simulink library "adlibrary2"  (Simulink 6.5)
undefined symbols (not defined in the file or in its folder): adlibrary2, ADM, DDRII, II, no_bitstream, SRAM, SX, XP, XRC
libraries: xbsIndex_r4 x360, adlibrary2 x9, adlibrary2_d2sram_0 x5, adlibrary2_ddr2dram_1 x4, adlibrary2_ddr_xpi0 x4, adlibrary2_ddr_xpl x3, adlibrary2_xpl32 x1, adlibrary2_xpl64 x1, adlibrary2_zbt64 x1, adlibrary2_zbt4_0 x1, adlibrary2_zbt4_1 x1, adlibrary2_zbt4_2 x1
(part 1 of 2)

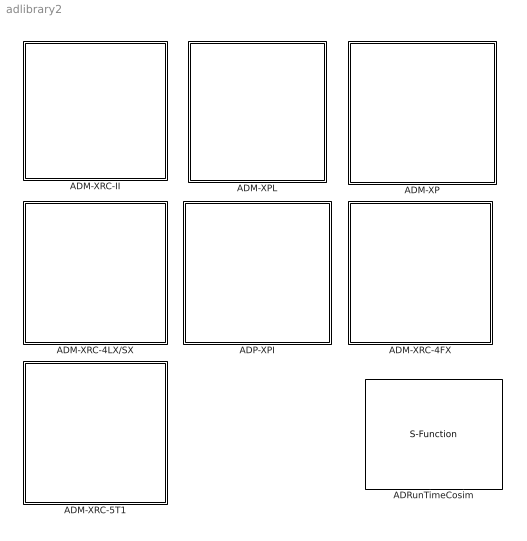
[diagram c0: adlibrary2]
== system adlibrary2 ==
  ADM-XP : Subsystem
  ADM-XPL : Subsystem
  ADM-XRC-4FX : Subsystem  AncestorBlock=adlibrary2/ADM-XRC-4LX//SX
  ADM-XRC-4LX/SX : Subsystem  AncestorBlock=adlibrary2/ADM-XRC-II
  ADM-XRC-5T1 : Subsystem  AncestorBlock=adlibrary2/ADM-XRC-4FX
  ADM-XRC-II : Subsystem
  ADP-XPI : Subsystem
  ADRunTimeCosim : S-Function  FunctionName=adcosim  Parameters='',index,bitstream,freq,single_step,shared  mask{index=0, bitstream=no_bitstream, freq=50, single_step=off, shared=None}
      mask prompts: index "Card Index"; freq "Clock Frequency"; single_step "Single Step"; shared "Share Access"

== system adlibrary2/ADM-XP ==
  DDR SDRAM 0 : Subsystem  mask{memsize=1}
      mask prompts: memsize "Simulation RAM Size (Mb)"
  DDR SDRAM 1 : Subsystem  mask{memsize=1}
      mask prompts: memsize "Simulation RAM Size (Mb)"
  DDRII SRAM 0 : Subsystem  mask{rate=1}
      mask prompts: rate "Simulink Clock Period"
  DDRII SRAM 1 : Subsystem  AncestorBlock=adlibrary2/ADM-XP/DDRII SRAM 0  mask{rate=1}
      mask prompts: rate "Simulink Clock Period"
  DDRII SRAM 2 : Subsystem  mask{rate=1}
      mask prompts: rate "Simulink Clock Period"
  DDRII SRAM 3 : Subsystem  mask{rate=1}
      mask prompts: rate "Simulink Clock Period"
  XPL 32 Bit Interface : adlibrary2/ADM-XPL/XPL 32 Bit Interface  SystemSampleTime=-1  program='load myprogram.txt'  clock_ratio=1.5  sstep_clk_sel_default=0
  XPL 64 Bit Interface : adlibrary2/ADM-XPL/XPL 64 Bit Interface  SystemSampleTime=-1  program='load myprogram.txt'  clock_ratio=1.5  sstep_clk_sel_default=0

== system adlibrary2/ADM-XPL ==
  DDR SDRAM : Subsystem  mask{memsize=1}
      mask prompts: memsize "Simulation RAM Size (Mb)"
  XPL 32 Bit Interface : Subsystem  mask{program='load myprogram.txt', clock_ratio=1.5, sstep_clk_sel_default=0}
      mask prompts: program "Local Bus Script Program"; clock_ratio "Clock Ratio"
  XPL 64 Bit Interface : Subsystem  mask{program='load myprogram.txt', clock_ratio=1.5, sstep_clk_sel_default=0}
      mask prompts: program "Local Bus Script Program"; clock_ratio "Clock Ratio"
  ZBT SRAM 64 : Subsystem  mask{rate=1}
      mask prompts: rate "Simulink Clock Period"

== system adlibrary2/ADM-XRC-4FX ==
  DDRII DRAM 0 : Subsystem  mask{rate=1}
      mask prompts: rate "Simulink Clock Period"
  DDRII DRAM 1 : Subsystem  mask{rate=1}
      mask prompts: rate "Simulink Clock Period"
  DDRII DRAM 2 : Subsystem  mask{rate=1}
      mask prompts: rate "Simulink Clock Period"
  DDRII DRAM 3 : Subsystem  mask{rate=1}
      mask prompts: rate "Simulink Clock Period"
  XPL 32 Bit Interface : adlibrary2/ADM-XPL/XPL 32 Bit Interface  SystemSampleTime=-1  program='load myprogram.txt'  clock_ratio=1.5  sstep_clk_sel_default=0
  XPL 64 Bit Interface : adlibrary2/ADM-XPL/XPL 64 Bit Interface  SystemSampleTime=-1  program='load myprogram.txt'  clock_ratio=1.5  sstep_clk_sel_default=0

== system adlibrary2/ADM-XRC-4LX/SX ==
  PLX 32 Bit Interface : adlibrary2/ADM-XRC-II/PLX 32 Bit Interface  SystemSampleTime=-1  program='load myprogram.txt'  clock_ratio=1.5  sstep_clk_sel_default=0
  ZBT SRAM 0 : Subsystem
  ZBT SRAM 1 : Subsystem
  ZBT SRAM 2 : Subsystem
  ZBT SRAM 3 : Subsystem
  ZBT SRAM 4 : Subsystem
  ZBT SRAM 5 : Subsystem

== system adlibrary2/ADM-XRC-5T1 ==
  DDRII DRAM 0 : Subsystem  mask{rate=1}
      mask prompts: rate "Simulink Clock Period"
  DDRII DRAM 1 : Subsystem  mask{rate=1}
      mask prompts: rate "Simulink Clock Period"
  XPL 32 Bit Interface : adlibrary2/ADM-XPL/XPL 32 Bit Interface  SystemSampleTime=-1  program='load myprogram.txt'  clock_ratio=1.5  sstep_clk_sel_default=0
  XPL 64 Bit Interface : adlibrary2/ADM-XPL/XPL 64 Bit Interface  SystemSampleTime=-1  program='load myprogram.txt'  clock_ratio=1.5  sstep_clk_sel_default=0

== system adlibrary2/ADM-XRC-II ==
  PLX 32 Bit Interface : Subsystem  mask{program='load myprogram.txt', clock_ratio=1.5, sstep_clk_sel_default=0}
      mask prompts: program "Local Bus Script Program"; clock_ratio "Clock Ratio"
  "XRM DDR SDRAM " : Subsystem  mask{memsize=1}
      mask prompts: memsize "Simulation RAM Size (Mb)"
  ZBT SRAM 0 : Subsystem  mask{rate=1}
      mask prompts: rate "Simulink Clock Period"
  ZBT SRAM 1 : Subsystem  mask{rate=1}
      mask prompts: rate "Simulink Clock Period"
  ZBT SRAM 2 : Subsystem  mask{rate=1}
      mask prompts: rate "Simulink Clock Period"
  ZBT SRAM 3 : Subsystem  mask{rate=1}
      mask prompts: rate "Simulink Clock Period"
  ZBT SRAM 4 : Subsystem  mask{rate=1}
      mask prompts: rate "Simulink Clock Period"
  ZBT SRAM 5 : Subsystem  mask{rate=1}
      mask prompts: rate "Simulink Clock Period:"

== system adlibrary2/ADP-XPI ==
  DDR SDRAM 0 : Subsystem  mask{memsize=1}
      mask prompts: memsize "Simulation RAM Size (Mb)"
  DDR SDRAM 1 : Subsystem  mask{memsize=1}
      mask prompts: memsize "Simulation RAM Size (Mb)"
  DDR SDRAM 2 : Subsystem  mask{memsize=1}
      mask prompts: memsize "Simulation RAM Size (Mb)"
  DDR SDRAM 3 : Subsystem  mask{memsize=1}
      mask prompts: memsize "Simulation RAM Size (Mb)"
  DDRII SRAM 0 : Subsystem
  XPL 32 Bit Interface : adlibrary2/ADM-XPL/XPL 32 Bit Interface  SystemSampleTime=-1  program='load myprogram.txt'  clock_ratio=1.5  sstep_clk_sel_default=0
  XPL 64 Bit Interface : adlibrary2/ADM-XPL/XPL 64 Bit Interface  SystemSampleTime=-1  program='load myprogram.txt'  clock_ratio=1.5  sstep_clk_sel_default=0

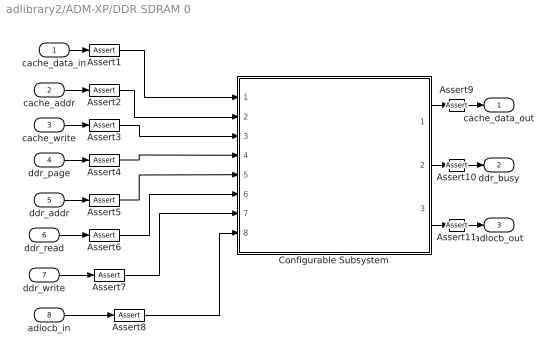
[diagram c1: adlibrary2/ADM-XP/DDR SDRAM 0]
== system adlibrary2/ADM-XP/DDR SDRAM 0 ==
  cache_data_in : Inport
  cache_addr : Inport  Port=2
  cache_write : Inport  Port=3
  ddr_page : Inport  Port=4
  ddr_addr : Inport  Port=5
  ddr_read : Inport  Port=6
  ddr_write : Inport  Port=7
  adlocb_in : Inport  Port=8
  Assert{1..11} (11 alike) : xbsIndex_r4/Assert  assert_type=off  type_source=Explicitly  arith_type="Signed  (2's comp)"  n_bits=16  bin_pt=14  assert_rate=on  rate_source=Explicitly  period=ad_get_simulink_period  output_port=on  block_type=assert
  Configurable Subsystem : Subsystem  Tag=configX  BlockChoice=DDR SDRAM 32bit Simulation  mask{memsize=memsize}
      mask prompts: memsize "Simulation Ram Size (Mb)"
  cache_data_out : Outport
  ddr_busy : Outport  Port=2
  adlocb_out : Outport  Port=3
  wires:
  Configurable Subsystem/3(adlocb_out) -> Assert11/1
  Configurable Subsystem/2(ddr_busy) -> Assert10/1
  Configurable Subsystem/1(cache_data_out) -> Assert9/1
  cache_data_in/1 -> Assert1/1
  cache_addr/1 -> Assert2/1
  cache_write/1 -> Assert3/1
  ddr_page/1 -> Assert4/1
  ddr_addr/1 -> Assert5/1
  ddr_read/1 -> Assert6/1
  ddr_write/1 -> Assert7/1
  adlocb_in/1 -> Assert8/1
  Assert1/1 -> Configurable Subsystem/1(cache_data_in)
  Assert2/1 -> Configurable Subsystem/2(cache_addr)
  Assert3/1 -> Configurable Subsystem/3(cache_write)
  Assert4/1 -> Configurable Subsystem/4(ddr_page)
  Assert5/1 -> Configurable Subsystem/5(ddr_addr)
  Assert6/1 -> Configurable Subsystem/6(ddr_read)
  Assert7/1 -> Configurable Subsystem/7(ddr_write)
  Assert8/1 -> Configurable Subsystem/8(adlocb_in)
  Assert9/1 -> cache_data_out/1
  Assert10/1 -> ddr_busy/1
  Assert11/1 -> adlocb_out/1

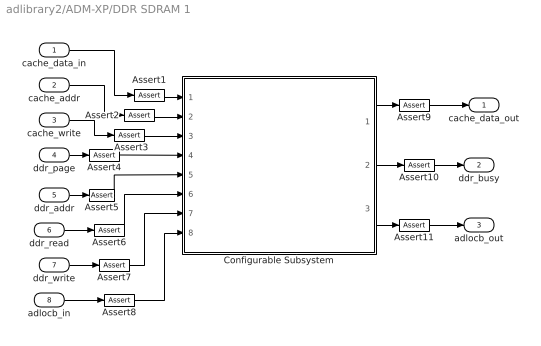
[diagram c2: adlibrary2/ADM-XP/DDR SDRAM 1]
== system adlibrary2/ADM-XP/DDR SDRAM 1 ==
  cache_data_in : Inport
  cache_addr : Inport  Port=2
  cache_write : Inport  Port=3
  ddr_page : Inport  Port=4
  ddr_addr : Inport  Port=5
  ddr_read : Inport  Port=6
  ddr_write : Inport  Port=7
  adlocb_in : Inport  Port=8
  Assert{1..11} (11 alike) : xbsIndex_r4/Assert  assert_type=off  type_source=Explicitly  arith_type="Signed  (2's comp)"  n_bits=16  bin_pt=14  assert_rate=on  rate_source=Explicitly  period=ad_get_simulink_period  output_port=on  block_type=assert
  Configurable Subsystem : Subsystem  Tag=configX  BlockChoice=DDR SDRAM 32bit Simulation  mask{memsize=memsize}
      mask prompts: memsize "Simulation Ram Size (Mb)"
  cache_data_out : Outport
  ddr_busy : Outport  Port=2
  adlocb_out : Outport  Port=3
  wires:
  Configurable Subsystem/3(adlocb_out) -> Assert11/1
  Configurable Subsystem/2(ddr_busy) -> Assert10/1
  Configurable Subsystem/1(cache_data_out) -> Assert9/1
  cache_data_in/1 -> Assert1/1
  cache_addr/1 -> Assert2/1
  cache_write/1 -> Assert3/1
  ddr_page/1 -> Assert4/1
  ddr_addr/1 -> Assert5/1
  ddr_read/1 -> Assert6/1
  ddr_write/1 -> Assert7/1
  adlocb_in/1 -> Assert8/1
  Assert1/1 -> Configurable Subsystem/1(cache_data_in)
  Assert2/1 -> Configurable Subsystem/2(cache_addr)
  Assert3/1 -> Configurable Subsystem/3(cache_write)
  Assert4/1 -> Configurable Subsystem/4(ddr_page)
  Assert5/1 -> Configurable Subsystem/5(ddr_addr)
  Assert6/1 -> Configurable Subsystem/6(ddr_read)
  Assert7/1 -> Configurable Subsystem/7(ddr_write)
  Assert8/1 -> Configurable Subsystem/8(adlocb_in)
  Assert9/1 -> cache_data_out/1
  Assert10/1 -> ddr_busy/1
  Assert11/1 -> adlocb_out/1

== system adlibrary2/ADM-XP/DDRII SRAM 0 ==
  d : Inport
  a : Inport  Port=2
  w : Inport  Port=3
  r : Inport  Port=4
  be : Inport  Port=5
  adlocb_in : Inport  Port=6
  Assert{1..9} (9 alike) : xbsIndex_r4/Assert  assert_type=off  type_source=Explicitly  arith_type="Signed  (2's comp)"  n_bits=16  bin_pt=14  assert_rate=on  rate_source=Explicitly  period=ad_get_simulink_period  output_port=on  block_type=assert
  Configurable Subsystem : Subsystem  Tag=configX  BlockChoice=DDRII SRAM Simulation
  q : Outport
  qv : Outport  Port=2
  adlocb_out : Outport  Port=3
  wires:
  Configurable Subsystem/1(q) -> Assert7/1
  d/1 -> Assert1/1
  a/1 -> Assert2/1
  w/1 -> Assert3/1
  r/1 -> Assert4/1
  be/1 -> Assert5/1
  adlocb_in/1 -> Assert6/1
  Configurable Subsystem/3(adlocb_out) -> Assert9/1
  Configurable Subsystem/2(qv) -> Assert8/1
  Assert1/1 -> Configurable Subsystem/1(d)
  Assert2/1 -> Configurable Subsystem/2(a)
  Assert3/1 -> Configurable Subsystem/3(w)
  Assert4/1 -> Configurable Subsystem/4(r)
  Assert5/1 -> Configurable Subsystem/5(be)
  Assert6/1 -> Configurable Subsystem/6(adlocb_in)
  Assert7/1 -> q/1
  Assert8/1 -> qv/1
  Assert9/1 -> adlocb_out/1

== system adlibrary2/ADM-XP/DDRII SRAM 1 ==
  d : Inport
  a : Inport  Port=2
  w : Inport  Port=3
  r : Inport  Port=4
  be : Inport  Port=5
  adlocb_in : Inport  Port=6
  Assert{1..9} (9 alike) : xbsIndex_r4/Assert  assert_type=off  type_source=Explicitly  arith_type="Signed  (2's comp)"  n_bits=16  bin_pt=14  assert_rate=on  rate_source=Explicitly  period=ad_get_simulink_period  output_port=on  block_type=assert
  Configurable Subsystem : Subsystem  Tag=configX  BlockChoice=DDRII SRAM Simulation
  q : Outport
  qv : Outport  Port=2
  adlocb_out : Outport  Port=3
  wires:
  Configurable Subsystem/1(q) -> Assert7/1
  d/1 -> Assert1/1
  a/1 -> Assert2/1
  w/1 -> Assert3/1
  r/1 -> Assert4/1
  be/1 -> Assert5/1
  adlocb_in/1 -> Assert6/1
  Configurable Subsystem/3(adlocb_out) -> Assert9/1
  Configurable Subsystem/2(qv) -> Assert8/1
  Assert1/1 -> Configurable Subsystem/1(d)
  Assert2/1 -> Configurable Subsystem/2(a)
  Assert3/1 -> Configurable Subsystem/3(w)
  Assert4/1 -> Configurable Subsystem/4(r)
  Assert5/1 -> Configurable Subsystem/5(be)
  Assert6/1 -> Configurable Subsystem/6(adlocb_in)
  Assert7/1 -> q/1
  Assert8/1 -> qv/1
  Assert9/1 -> adlocb_out/1

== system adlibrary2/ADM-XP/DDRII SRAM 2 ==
  d : Inport
  a : Inport  Port=2
  w : Inport  Port=3
  r : Inport  Port=4
  be : Inport  Port=5
  adlocb_in : Inport  Port=6
  Assert{1..9} (9 alike) : xbsIndex_r4/Assert  assert_type=off  type_source=Explicitly  arith_type="Signed  (2's comp)"  n_bits=16  bin_pt=14  assert_rate=on  rate_source=Explicitly  period=ad_get_simulink_period  output_port=on  block_type=assert
  Configurable Subsystem : Subsystem  Tag=configX  BlockChoice=DDRII SRAM Simulation
  q : Outport
  qv : Outport  Port=2
  adlocb_out : Outport  Port=3
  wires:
  Configurable Subsystem/2(qv) -> Assert8/1
  Configurable Subsystem/3(adlocb_out) -> Assert9/1
  adlocb_in/1 -> Assert6/1
  be/1 -> Assert5/1
  r/1 -> Assert4/1
  w/1 -> Assert3/1
  a/1 -> Assert2/1
  d/1 -> Assert1/1
  Configurable Subsystem/1(q) -> Assert7/1
  Assert7/1 -> q/1
  Assert8/1 -> qv/1
  Assert9/1 -> adlocb_out/1
  Assert1/1 -> Configurable Subsystem/1(d)
  Assert2/1 -> Configurable Subsystem/2(a)
  Assert3/1 -> Configurable Subsystem/3(w)
  Assert4/1 -> Configurable Subsystem/4(r)
  Assert5/1 -> Configurable Subsystem/5(be)
  Assert6/1 -> Configurable Subsystem/6(adlocb_in)

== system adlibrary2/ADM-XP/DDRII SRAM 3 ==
  d : Inport
  a : Inport  Port=2
  w : Inport  Port=3
  r : Inport  Port=4
  be : Inport  Port=5
  adlocb_in : Inport  Port=6
  Assert{1..9} (9 alike) : xbsIndex_r4/Assert  assert_type=off  type_source=Explicitly  arith_type="Signed  (2's comp)"  n_bits=16  bin_pt=14  assert_rate=on  rate_source=Explicitly  period=ad_get_simulink_period  output_port=on  block_type=assert
  Configurable Subsystem : Subsystem  Tag=configX  BlockChoice=DDRII SRAM Simulation
  q : Outport
  qv : Outport  Port=2
  adlocb_out : Outport  Port=3
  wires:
  Configurable Subsystem/2(qv) -> Assert8/1
  Configurable Subsystem/3(adlocb_out) -> Assert9/1
  adlocb_in/1 -> Assert6/1
  be/1 -> Assert5/1
  r/1 -> Assert4/1
  w/1 -> Assert3/1
  a/1 -> Assert2/1
  d/1 -> Assert1/1
  Configurable Subsystem/1(q) -> Assert7/1
  Assert1/1 -> Configurable Subsystem/1(d)
  Assert2/1 -> Configurable Subsystem/2(a)
  Assert3/1 -> Configurable Subsystem/3(w)
  Assert4/1 -> Configurable Subsystem/4(r)
  Assert5/1 -> Configurable Subsystem/5(be)
  Assert6/1 -> Configurable Subsystem/6(adlocb_in)
  Assert7/1 -> q/1
  Assert8/1 -> qv/1
  Assert9/1 -> adlocb_out/1

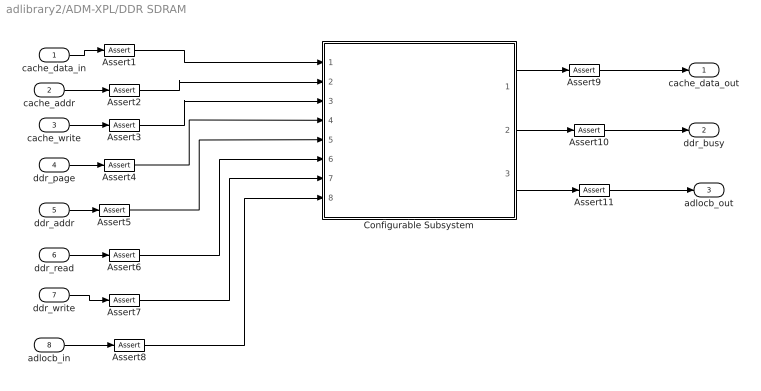
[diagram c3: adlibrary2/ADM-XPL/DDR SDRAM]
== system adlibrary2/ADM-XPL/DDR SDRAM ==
  cache_data_in : Inport
  cache_addr : Inport  Port=2
  cache_write : Inport  Port=3
  ddr_page : Inport  Port=4
  ddr_addr : Inport  Port=5
  ddr_read : Inport  Port=6
  ddr_write : Inport  Port=7
  adlocb_in : Inport  Port=8
  Assert{1..11} (11 alike) : xbsIndex_r4/Assert  assert_type=off  type_source=Explicitly  arith_type="Signed  (2's comp)"  n_bits=16  bin_pt=14  assert_rate=on  rate_source=Explicitly  period=ad_get_simulink_period  output_port=on  block_type=assert
  Configurable Subsystem : Subsystem  Tag=configX  BlockChoice=DDR SDRAM 32bit Simulation  mask{memsize=memsize}
      mask prompts: memsize "Simulation Ram Size (Mb)"
  cache_data_out : Outport
  ddr_busy : Outport  Port=2
  adlocb_out : Outport  Port=3
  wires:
  cache_data_in/1 -> Assert1/1
  cache_addr/1 -> Assert2/1
  cache_write/1 -> Assert3/1
  ddr_page/1 -> Assert4/1
  ddr_addr/1 -> Assert5/1
  ddr_read/1 -> Assert6/1
  ddr_write/1 -> Assert7/1
  adlocb_in/1 -> Assert8/1
  Configurable Subsystem/1(cache_data_out) -> Assert9/1
  Configurable Subsystem/2(ddr_busy) -> Assert10/1
  Configurable Subsystem/3(adlocb_out) -> Assert11/1
  Assert1/1 -> Configurable Subsystem/1(cache_data_in)
  Assert2/1 -> Configurable Subsystem/2(cache_addr)
  Assert3/1 -> Configurable Subsystem/3(cache_write)
  Assert4/1 -> Configurable Subsystem/4(ddr_page)
  Assert5/1 -> Configurable Subsystem/5(ddr_addr)
  Assert6/1 -> Configurable Subsystem/6(ddr_read)
  Assert7/1 -> Configurable Subsystem/7(ddr_write)
  Assert8/1 -> Configurable Subsystem/8(adlocb_in)
  Assert9/1 -> cache_data_out/1
  Assert10/1 -> ddr_busy/1
  Assert11/1 -> adlocb_out/1

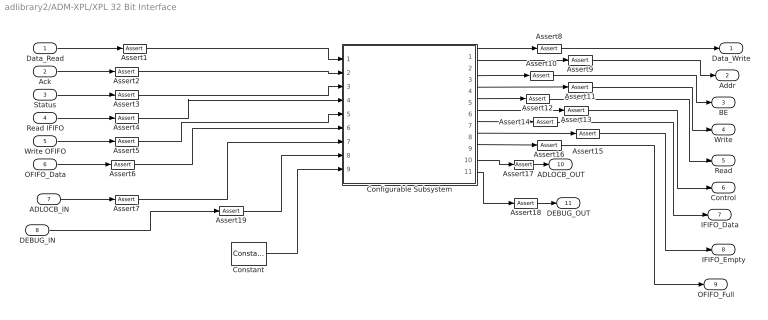
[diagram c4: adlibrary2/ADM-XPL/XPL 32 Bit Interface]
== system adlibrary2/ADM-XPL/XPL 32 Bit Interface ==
  Data_Read : Inport
  Ack : Inport  Port=2
  Status : Inport  Port=3
  Read IFIFO : Inport  Port=4
  Write OFIFO : Inport  Port=5
  OFIFO_Data : Inport  Port=6
  ADLOCB_IN : Inport  Port=7
  DEBUG_IN : Inport  Port=8
  Assert{1..19} (19 alike) : xbsIndex_r4/Assert  assert_type=off  type_source=Explicitly  arith_type="Signed  (2's comp)"  n_bits=16  bin_pt=14  assert_rate=on  rate_source=Explicitly  period=ad_get_simulink_period  output_port=on  block_type=assert
  Configurable Subsystem : Subsystem  Tag=configX  BlockChoice=XPL 32Bit Simulation  mask{program=program, clock_ratio=clock_ratio}
      mask prompts: program "Local Bus Script Program"; clock_ratio "Clock Ratio"
  Constant : xbsIndex_r4/Constant  arith_type=Boolean  const=sstep_clk_sel_default  n_bits=16  bin_pt=14  explicit_period=on  period=ad_get_simulink_period  equ=P=C  opselect=C  inp2=PCIN>>17  opr=+  inp1=P  carry=CIN  dbl_ovrd=off  block_type=constant
  Data_Write : Outport
  Addr : Outport  Port=2
  BE : Outport  Port=3
  Write : Outport  Port=4
  Read : Outport  Port=5
  Control : Outport  Port=6
  IFIFO_Data : Outport  Port=7
  IFIFO_Empty : Outport  Port=8
  OFIFO_Full : Outport  Port=9
  ADLOCB_OUT : Outport  Port=10
  DEBUG_OUT : Outport  Port=11
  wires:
  Status/1 -> Assert3/1
  Ack/1 -> Assert2/1
  Data_Read/1 -> Assert1/1
  Configurable Subsystem/9(OFIFO_Full) -> Assert16/1
  Configurable Subsystem/8(IFIFO_Empty) -> Assert15/1
  Configurable Subsystem/7(IFIFO_Data) -> Assert14/1
  Configurable Subsystem/6(Control) -> Assert13/1
  Configurable Subsystem/5(Read) -> Assert12/1
  Configurable Subsystem/4(Write) -> Assert11/1
  Configurable Subsystem/3(BE) -> Assert10/1
  Configurable Subsystem/1(Data_Write) -> Assert8/1
  Configurable Subsystem/2(Addr) -> Assert9/1
  Read IFIFO/1 -> Assert4/1
  Write OFIFO/1 -> Assert5/1
  OFIFO_Data/1 -> Assert6/1
  ADLOCB_IN/1 -> Assert7/1
  Configurable Subsystem/10(ADLOCB_OUT) -> Assert17/1
  Assert1/1 -> Configurable Subsystem/1(Data_Read)
  Assert2/1 -> Configurable Subsystem/2(Ack)
  Assert3/1 -> Configurable Subsystem/3(Status)
  Assert4/1 -> Configurable Subsystem/4(Read IFIFO)
  Assert8/1 -> Data_Write/1
  Assert9/1 -> Addr/1
  Assert10/1 -> BE/1
  Assert11/1 -> Write/1
  Assert12/1 -> Read/1
  Assert13/1 -> Control/1
  Assert14/1 -> IFIFO_Data/1
  Assert15/1 -> IFIFO_Empty/1
  Assert16/1 -> OFIFO_Full/1
  Assert17/1 -> ADLOCB_OUT/1
  Assert5/1 -> Configurable Subsystem/5(Write OFIFO)
  Assert6/1 -> Configurable Subsystem/6(OFIFO_Data)
  Assert7/1 -> Configurable Subsystem/7(ADLOCB_IN)
  DEBUG_IN/1 -> Assert19/1
  Assert19/1 -> Configurable Subsystem/8(DEBUG_IN)
  Assert18/1 -> DEBUG_OUT/1
  Configurable Subsystem/11(DEBUG_OUT) -> Assert18/1
  Constant/1 -> Configurable Subsystem/9(sstep_clk_sel_default)

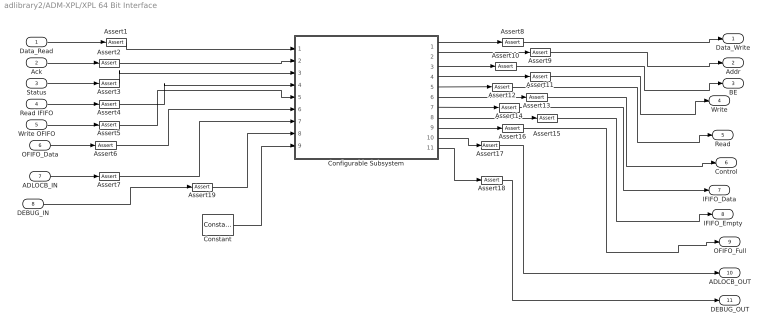
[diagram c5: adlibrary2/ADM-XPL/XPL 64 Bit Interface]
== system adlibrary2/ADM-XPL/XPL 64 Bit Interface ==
  Data_Read : Inport
  Ack : Inport  Port=2
  Status : Inport  Port=3
  Read IFIFO : Inport  Port=4
  Write OFIFO : Inport  Port=5
  OFIFO_Data : Inport  Port=6
  ADLOCB_IN : Inport  Port=7
  DEBUG_IN : Inport  Port=8
  Assert{1..19} (19 alike) : xbsIndex_r4/Assert  assert_type=off  type_source=Explicitly  arith_type="Signed  (2's comp)"  n_bits=16  bin_pt=14  assert_rate=on  rate_source=Explicitly  period=ad_get_simulink_period  output_port=on  block_type=assert
  Configurable Subsystem : Subsystem  Tag=configX  BlockChoice=XPL 64Bit Simulation  mask{program=program, clock_ratio=clock_ratio}
      mask prompts: program "Local Bus Script Program"; clock_ratio "Clock Ratio"
  Constant : xbsIndex_r4/Constant  arith_type=Boolean  const=sstep_clk_sel_default  n_bits=16  bin_pt=14  explicit_period=on  period=ad_get_simulink_period  equ=P=C  opselect=C  inp2=PCIN>>17  opr=+  inp1=P  carry=CIN  dbl_ovrd=off  block_type=constant
  Data_Write : Outport
  Addr : Outport  Port=2
  BE : Outport  Port=3
  Write : Outport  Port=4
  Read : Outport  Port=5
  Control : Outport  Port=6
  IFIFO_Data : Outport  Port=7
  IFIFO_Empty : Outport  Port=8
  OFIFO_Full : Outport  Port=9
  ADLOCB_OUT : Outport  Port=10
  DEBUG_OUT : Outport  Port=11
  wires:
  Status/1 -> Assert3/1
  Ack/1 -> Assert2/1
  Data_Read/1 -> Assert1/1
  Read IFIFO/1 -> Assert4/1
  Write OFIFO/1 -> Assert5/1
  OFIFO_Data/1 -> Assert6/1
  ADLOCB_IN/1 -> Assert7/1
  Assert1/1 -> Configurable Subsystem/1(Data_Read)
  Assert2/1 -> Configurable Subsystem/2(Ack)
  Assert3/1 -> Configurable Subsystem/3(Status)
  Assert4/1 -> Configurable Subsystem/4(Read IFIFO)
  Assert5/1 -> Configurable Subsystem/5(Write OFIFO)
  Assert6/1 -> Configurable Subsystem/6(OFIFO_Data)
  Assert7/1 -> Configurable Subsystem/7(ADLOCB_IN)
  DEBUG_IN/1 -> Assert19/1
  Assert19/1 -> Configurable Subsystem/8(DEBUG_IN)
  Constant/1 -> Configurable Subsystem/9(sstep_clk_sel_default)
  Configurable Subsystem/9(OFIFO_Full) -> Assert16/1
  Configurable Subsystem/8(IFIFO_Empty) -> Assert15/1
  Configurable Subsystem/7(IFIFO_Data) -> Assert14/1
  Configurable Subsystem/6(Control) -> Assert13/1
  Configurable Subsystem/5(Read) -> Assert12/1
  Configurable Subsystem/4(Write) -> Assert11/1
  Configurable Subsystem/3(BE) -> Assert10/1
  Configurable Subsystem/1(Data_Write) -> Assert8/1
  Configurable Subsystem/2(Addr) -> Assert9/1
  Configurable Subsystem/10(ADLOCB_OUT) -> Assert17/1
  Assert8/1 -> Data_Write/1
  Assert9/1 -> Addr/1
  Assert10/1 -> BE/1
  Assert11/1 -> Write/1
  Assert12/1 -> Read/1
  Assert13/1 -> Control/1
  Assert14/1 -> IFIFO_Data/1
  Assert15/1 -> IFIFO_Empty/1
  Assert16/1 -> OFIFO_Full/1
  Assert17/1 -> ADLOCB_OUT/1
  Assert18/1 -> DEBUG_OUT/1
  Configurable Subsystem/11(DEBUG_OUT) -> Assert18/1

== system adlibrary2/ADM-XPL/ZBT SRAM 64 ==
  d : Inport
  a : Inport  Port=2
  w : Inport  Port=3
  r : Inport  Port=4
  be : Inport  Port=5
  adlocb_in : Inport  Port=6
  Assert{1..9} (9 alike) : xbsIndex_r4/Assert  assert_type=off  type_source=Explicitly  arith_type="Signed  (2's comp)"  n_bits=16  bin_pt=14  assert_rate=on  rate_source=Explicitly  period=ad_get_simulink_period  output_port=on  block_type=assert
  Configurable Subsystem : Subsystem  Tag=configX  BlockChoice=ZBT SRAM 64bit Simulation
  q : Outport
  qv : Outport  Port=2
  adlocb_out : Outport  Port=3
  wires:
  d/1 -> Assert1/1
  a/1 -> Assert2/1
  w/1 -> Assert3/1
  r/1 -> Assert4/1
  be/1 -> Assert5/1
  adlocb_in/1 -> Assert6/1
  Configurable Subsystem/1(q) -> Assert7/1
  Configurable Subsystem/2(qv) -> Assert8/1
  Configurable Subsystem/3(adlocb_out) -> Assert9/1
  Assert1/1 -> Configurable Subsystem/1(d)
  Assert2/1 -> Configurable Subsystem/2(a)
  Assert3/1 -> Configurable Subsystem/3(w)
  Assert4/1 -> Configurable Subsystem/4(r)
  Assert5/1 -> Configurable Subsystem/5(be)
  Assert6/1 -> Configurable Subsystem/6(adlocb_in)
  Assert7/1 -> q/1
  Assert8/1 -> qv/1
  Assert9/1 -> adlocb_out/1

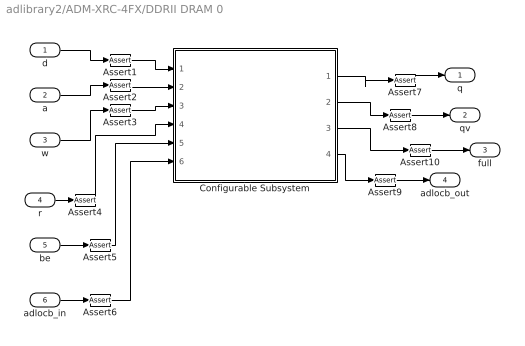
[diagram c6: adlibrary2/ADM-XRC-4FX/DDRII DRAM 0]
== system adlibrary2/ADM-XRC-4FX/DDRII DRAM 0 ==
  d : Inport
  a : Inport  Port=2
  w : Inport  Port=3
  r : Inport  Port=4
  be : Inport  Port=5
  adlocb_in : Inport  Port=6
  Assert{1..10} (10 alike) : xbsIndex_r4/Assert  assert_type=off  type_source=Explicitly  arith_type="Signed  (2's comp)"  n_bits=16  bin_pt=14  assert_rate=on  rate_source=Explicitly  period=ad_get_simulink_period  output_port=on  block_type=assert
  Configurable Subsystem : Subsystem  Tag=configX  BlockChoice=DDRII DRAM Simulation
  q : Outport
  qv : Outport  Port=2
  full : Outport  Port=3
  adlocb_out : Outport  Port=4
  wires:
  Assert9/1 -> adlocb_out/1
  Assert8/1 -> qv/1
  Assert7/1 -> q/1
  Assert6/1 -> Configurable Subsystem/6(adlocb_in)
  Assert5/1 -> Configurable Subsystem/5(be)
  Assert4/1 -> Configurable Subsystem/4(r)
  Assert3/1 -> Configurable Subsystem/3(w)
  Assert2/1 -> Configurable Subsystem/2(a)
  Assert1/1 -> Configurable Subsystem/1(d)
  Configurable Subsystem/2(qv) -> Assert8/1
  Configurable Subsystem/4(adlocb_out) -> Assert9/1
  adlocb_in/1 -> Assert6/1
  be/1 -> Assert5/1
  r/1 -> Assert4/1
  w/1 -> Assert3/1
  a/1 -> Assert2/1
  d/1 -> Assert1/1
  Configurable Subsystem/1(q) -> Assert7/1
  Assert10/1 -> full/1
  Configurable Subsystem/3(full) -> Assert10/1

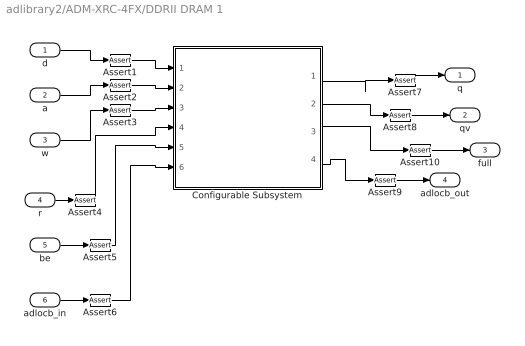
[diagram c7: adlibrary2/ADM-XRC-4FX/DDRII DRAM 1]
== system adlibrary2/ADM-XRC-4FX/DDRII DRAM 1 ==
  d : Inport
  a : Inport  Port=2
  w : Inport  Port=3
  r : Inport  Port=4
  be : Inport  Port=5
  adlocb_in : Inport  Port=6
  Assert{1..10} (10 alike) : xbsIndex_r4/Assert  assert_type=off  type_source=Explicitly  arith_type="Signed  (2's comp)"  n_bits=16  bin_pt=14  assert_rate=on  rate_source=Explicitly  period=ad_get_simulink_period  output_port=on  block_type=assert
  Configurable Subsystem : Subsystem  Tag=configX  BlockChoice=DDRII DRAM Generation
  q : Outport
  qv : Outport  Port=2
  full : Outport  Port=3
  adlocb_out : Outport  Port=4
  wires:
  Configurable Subsystem/3(full) -> Assert10/1
  Assert10/1 -> full/1
  Configurable Subsystem/1(q) -> Assert7/1
  d/1 -> Assert1/1
  a/1 -> Assert2/1
  w/1 -> Assert3/1
  r/1 -> Assert4/1
  be/1 -> Assert5/1
  adlocb_in/1 -> Assert6/1
  Configurable Subsystem/4(adlocb_out) -> Assert9/1
  Configurable Subsystem/2(qv) -> Assert8/1
  Assert1/1 -> Configurable Subsystem/1(d)
  Assert2/1 -> Configurable Subsystem/2(a)
  Assert3/1 -> Configurable Subsystem/3(w)
  Assert4/1 -> Configurable Subsystem/4(r)
  Assert5/1 -> Configurable Subsystem/5(be)
  Assert6/1 -> Configurable Subsystem/6(adlocb_in)
  Assert7/1 -> q/1
  Assert8/1 -> qv/1
  Assert9/1 -> adlocb_out/1

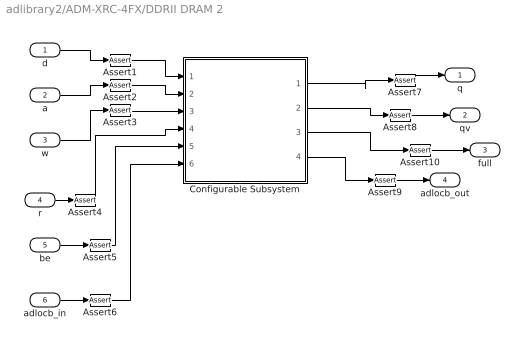
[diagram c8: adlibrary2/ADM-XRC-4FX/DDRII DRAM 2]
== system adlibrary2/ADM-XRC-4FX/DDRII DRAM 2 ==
  d : Inport
  a : Inport  Port=2
  w : Inport  Port=3
  r : Inport  Port=4
  be : Inport  Port=5
  adlocb_in : Inport  Port=6
  Assert{1..10} (10 alike) : xbsIndex_r4/Assert  assert_type=off  type_source=Explicitly  arith_type="Signed  (2's comp)"  n_bits=16  bin_pt=14  assert_rate=on  rate_source=Explicitly  period=ad_get_simulink_period  output_port=on  block_type=assert
  Configurable Subsystem : Subsystem  Tag=configX  BlockChoice=DDRII DRAM Generation
  q : Outport
  qv : Outport  Port=2
  full : Outport  Port=3
  adlocb_out : Outport  Port=4
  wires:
  Configurable Subsystem/3(full) -> Assert10/1
  Assert10/1 -> full/1
  Configurable Subsystem/1(q) -> Assert7/1
  d/1 -> Assert1/1
  a/1 -> Assert2/1
  w/1 -> Assert3/1
  r/1 -> Assert4/1
  be/1 -> Assert5/1
  adlocb_in/1 -> Assert6/1
  Configurable Subsystem/4(adlocb_out) -> Assert9/1
  Configurable Subsystem/2(qv) -> Assert8/1
  Assert1/1 -> Configurable Subsystem/1(d)
  Assert2/1 -> Configurable Subsystem/2(a)
  Assert3/1 -> Configurable Subsystem/3(w)
  Assert4/1 -> Configurable Subsystem/4(r)
  Assert5/1 -> Configurable Subsystem/5(be)
  Assert6/1 -> Configurable Subsystem/6(adlocb_in)
  Assert7/1 -> q/1
  Assert8/1 -> qv/1
  Assert9/1 -> adlocb_out/1

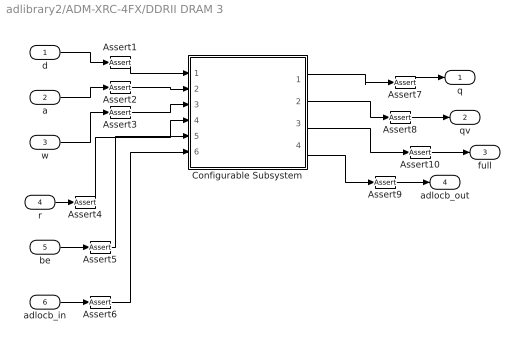
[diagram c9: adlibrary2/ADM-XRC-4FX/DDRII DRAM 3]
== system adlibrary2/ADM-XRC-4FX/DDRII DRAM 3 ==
  d : Inport
  a : Inport  Port=2
  w : Inport  Port=3
  r : Inport  Port=4
  be : Inport  Port=5
  adlocb_in : Inport  Port=6
  Assert{1..10} (10 alike) : xbsIndex_r4/Assert  assert_type=off  type_source=Explicitly  arith_type="Signed  (2's comp)"  n_bits=16  bin_pt=14  assert_rate=on  rate_source=Explicitly  period=ad_get_simulink_period  output_port=on  block_type=assert
  Configurable Subsystem : Subsystem  Tag=configX  BlockChoice=DDRII DRAM Generation
  q : Outport
  qv : Outport  Port=2
  full : Outport  Port=3
  adlocb_out : Outport  Port=4
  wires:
  Configurable Subsystem/3(full) -> Assert10/1
  Assert10/1 -> full/1
  Configurable Subsystem/1(q) -> Assert7/1
  d/1 -> Assert1/1
  a/1 -> Assert2/1
  w/1 -> Assert3/1
  r/1 -> Assert4/1
  be/1 -> Assert5/1
  adlocb_in/1 -> Assert6/1
  Configurable Subsystem/4(adlocb_out) -> Assert9/1
  Configurable Subsystem/2(qv) -> Assert8/1
  Assert1/1 -> Configurable Subsystem/1(d)
  Assert2/1 -> Configurable Subsystem/2(a)
  Assert3/1 -> Configurable Subsystem/3(w)
  Assert4/1 -> Configurable Subsystem/4(r)
  Assert5/1 -> Configurable Subsystem/5(be)
  Assert6/1 -> Configurable Subsystem/6(adlocb_in)
  Assert7/1 -> q/1
  Assert8/1 -> qv/1
  Assert9/1 -> adlocb_out/1

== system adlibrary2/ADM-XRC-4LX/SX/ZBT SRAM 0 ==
  d : Inport
  a : Inport  Port=2
  w : Inport  Port=3
  r : Inport  Port=4
  be : Inport  Port=5
  adlocb_in : Inport  Port=6
  Assert{1..9} (9 alike) : xbsIndex_r4/Assert  assert_type=off  type_source=Explicitly  arith_type="Signed  (2's comp)"  n_bits=16  bin_pt=14  assert_rate=on  rate_source=Explicitly  period=ad_get_simulink_period  output_port=on  block_type=assert
  Configurable Subsystem : Subsystem  Tag=configX  BlockChoice=ZBT SRAM 32Bit Simulation
  q : Outport
  qv : Outport  Port=2
  adlocb_out : Outport  Port=3
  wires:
  Configurable Subsystem/3(adlocb_out) -> Assert9/1
  Configurable Subsystem/2(qv) -> Assert8/1
  Configurable Subsystem/1(q) -> Assert7/1
  adlocb_in/1 -> Assert6/1
  be/1 -> Assert5/1
  r/1 -> Assert4/1
  w/1 -> Assert3/1
  a/1 -> Assert2/1
  d/1 -> Assert1/1
  Assert1/1 -> Configurable Subsystem/1(d)
  Assert2/1 -> Configurable Subsystem/2(a)
  Assert3/1 -> Configurable Subsystem/3(w)
  Assert4/1 -> Configurable Subsystem/4(r)
  Assert5/1 -> Configurable Subsystem/5(be)
  Assert6/1 -> Configurable Subsystem/6(adlocb_in)
  Assert7/1 -> q/1
  Assert8/1 -> qv/1
  Assert9/1 -> adlocb_out/1

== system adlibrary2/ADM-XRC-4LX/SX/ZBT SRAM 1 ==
  d : Inport
  a : Inport  Port=2
  w : Inport  Port=3
  r : Inport  Port=4
  be : Inport  Port=5
  adlocb_in : Inport  Port=6
  Assert{1..9} (9 alike) : xbsIndex_r4/Assert  assert_type=off  type_source=Explicitly  arith_type="Signed  (2's comp)"  n_bits=16  bin_pt=14  assert_rate=on  rate_source=Explicitly  period=ad_get_simulink_period  output_port=on  block_type=assert
  Configurable Subsystem : Subsystem  Tag=configX  BlockChoice=ZBT SRAM 32Bit Simulation
  q : Outport
  qv : Outport  Port=2
  adlocb_out : Outport  Port=3
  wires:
  d/1 -> Assert1/1
  a/1 -> Assert2/1
  w/1 -> Assert3/1
  r/1 -> Assert4/1
  be/1 -> Assert5/1
  adlocb_in/1 -> Assert6/1
  Configurable Subsystem/1(q) -> Assert7/1
  Configurable Subsystem/2(qv) -> Assert8/1
  Configurable Subsystem/3(adlocb_out) -> Assert9/1
  Assert1/1 -> Configurable Subsystem/1(d)
  Assert2/1 -> Configurable Subsystem/2(a)
  Assert3/1 -> Configurable Subsystem/3(w)
  Assert4/1 -> Configurable Subsystem/4(r)
  Assert5/1 -> Configurable Subsystem/5(be)
  Assert6/1 -> Configurable Subsystem/6(adlocb_in)
  Assert7/1 -> q/1
  Assert8/1 -> qv/1
  Assert9/1 -> adlocb_out/1

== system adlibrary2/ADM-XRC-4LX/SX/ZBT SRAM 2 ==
  d : Inport
  a : Inport  Port=2
  w : Inport  Port=3
  r : Inport  Port=4
  be : Inport  Port=5
  adlocb_in : Inport  Port=6
  Assert{1..9} (9 alike) : xbsIndex_r4/Assert  assert_type=off  type_source=Explicitly  arith_type="Signed  (2's comp)"  n_bits=16  bin_pt=14  assert_rate=on  rate_source=Explicitly  period=ad_get_simulink_period  output_port=on  block_type=assert
  Configurable Subsystem : Subsystem  Tag=configX  BlockChoice=ZBT SRAM 32Bit Simulation
  q : Outport
  qv : Outport  Port=2
  adlocb_out : Outport  Port=3
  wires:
  d/1 -> Assert1/1
  a/1 -> Assert2/1
  w/1 -> Assert3/1
  r/1 -> Assert4/1
  be/1 -> Assert5/1
  adlocb_in/1 -> Assert6/1
  Configurable Subsystem/1(q) -> Assert8/1
  Configurable Subsystem/2(qv) -> Assert9/1
  Configurable Subsystem/3(adlocb_out) -> Assert7/1
  Assert1/1 -> Configurable Subsystem/1(d)
  Assert2/1 -> Configurable Subsystem/2(a)
  Assert3/1 -> Configurable Subsystem/3(w)
  Assert4/1 -> Configurable Subsystem/4(r)
  Assert5/1 -> Configurable Subsystem/5(be)
  Assert6/1 -> Configurable Subsystem/6(adlocb_in)
  Assert7/1 -> adlocb_out/1
  Assert8/1 -> q/1
  Assert9/1 -> qv/1

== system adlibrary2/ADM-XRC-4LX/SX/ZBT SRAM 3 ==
  d : Inport
  a : Inport  Port=2
  w : Inport  Port=3
  r : Inport  Port=4
  be : Inport  Port=5
  adlocb_in : Inport  Port=6
  Assert{1..9} (9 alike) : xbsIndex_r4/Assert  assert_type=off  type_source=Explicitly  arith_type="Signed  (2's comp)"  n_bits=16  bin_pt=14  assert_rate=on  rate_source=Explicitly  period=ad_get_simulink_period  output_port=on  block_type=assert
  Configurable Subsystem : Subsystem  Tag=configX  BlockChoice=ZBT SRAM 32Bit Simulation
  q : Outport
  qv : Outport  Port=2
  adlocb_out : Outport  Port=3
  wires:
  d/1 -> Assert1/1
  a/1 -> Assert2/1
  w/1 -> Assert3/1
  r/1 -> Assert4/1
  be/1 -> Assert5/1
  adlocb_in/1 -> Assert6/1
  Configurable Subsystem/1(q) -> Assert7/1
  Configurable Subsystem/2(qv) -> Assert8/1
  Configurable Subsystem/3(adlocb_out) -> Assert9/1
  Assert1/1 -> Configurable Subsystem/1(d)
  Assert2/1 -> Configurable Subsystem/2(a)
  Assert3/1 -> Configurable Subsystem/3(w)
  Assert4/1 -> Configurable Subsystem/4(r)
  Assert5/1 -> Configurable Subsystem/5(be)
  Assert6/1 -> Configurable Subsystem/6(adlocb_in)
  Assert7/1 -> q/1
  Assert8/1 -> qv/1
  Assert9/1 -> adlocb_out/1

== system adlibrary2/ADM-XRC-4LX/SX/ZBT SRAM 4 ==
  d : Inport
  a : Inport  Port=2
  w : Inport  Port=3
  r : Inport  Port=4
  be : Inport  Port=5
  adlocb_in : Inport  Port=6
  Assert{1..9} (9 alike) : xbsIndex_r4/Assert  assert_type=off  type_source=Explicitly  arith_type="Signed  (2's comp)"  n_bits=16  bin_pt=14  assert_rate=on  rate_source=Explicitly  period=ad_get_simulink_period  output_port=on  block_type=assert
  Configurable Subsystem : Subsystem  Tag=configX  BlockChoice=ZBT SRAM 32Bit Simulation
  q : Outport
  qv : Outport  Port=2
  adlocb_out : Outport  Port=3
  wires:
  d/1 -> Assert1/1
  a/1 -> Assert2/1
  w/1 -> Assert3/1
  r/1 -> Assert4/1
  be/1 -> Assert5/1
  adlocb_in/1 -> Assert6/1
  Configurable Subsystem/1(q) -> Assert7/1
  Configurable Subsystem/2(qv) -> Assert8/1
  Configurable Subsystem/3(adlocb_out) -> Assert9/1
  Assert1/1 -> Configurable Subsystem/1(d)
  Assert2/1 -> Configurable Subsystem/2(a)
  Assert3/1 -> Configurable Subsystem/3(w)
  Assert4/1 -> Configurable Subsystem/4(r)
  Assert5/1 -> Configurable Subsystem/5(be)
  Assert6/1 -> Configurable Subsystem/6(adlocb_in)
  Assert7/1 -> q/1
  Assert8/1 -> qv/1
  Assert9/1 -> adlocb_out/1

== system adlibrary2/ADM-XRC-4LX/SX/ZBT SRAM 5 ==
  d : Inport
  a : Inport  Port=2
  w : Inport  Port=3
  r : Inport  Port=4
  be : Inport  Port=5
  adlocb_in : Inport  Port=6
  Assert{1..9} (9 alike) : xbsIndex_r4/Assert  assert_type=off  type_source=Explicitly  arith_type="Signed  (2's comp)"  n_bits=16  bin_pt=14  assert_rate=on  rate_source=Explicitly  period=ad_get_simulink_period  output_port=on  block_type=assert
  Configurable Subsystem : Subsystem  Tag=configX  BlockChoice=ZBT SRAM 32Bit Simulation
  q : Outport
  qv : Outport  Port=2
  adlocb_out : Outport  Port=3
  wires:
  d/1 -> Assert1/1
  a/1 -> Assert2/1
  w/1 -> Assert3/1
  r/1 -> Assert4/1
  be/1 -> Assert5/1
  adlocb_in/1 -> Assert6/1
  Configurable Subsystem/1(q) -> Assert7/1
  Configurable Subsystem/2(qv) -> Assert8/1
  Configurable Subsystem/3(adlocb_out) -> Assert9/1
  Assert1/1 -> Configurable Subsystem/1(d)
  Assert2/1 -> Configurable Subsystem/2(a)
  Assert3/1 -> Configurable Subsystem/3(w)
  Assert4/1 -> Configurable Subsystem/4(r)
  Assert5/1 -> Configurable Subsystem/5(be)
  Assert6/1 -> Configurable Subsystem/6(adlocb_in)
  Assert7/1 -> q/1
  Assert8/1 -> qv/1
  Assert9/1 -> adlocb_out/1

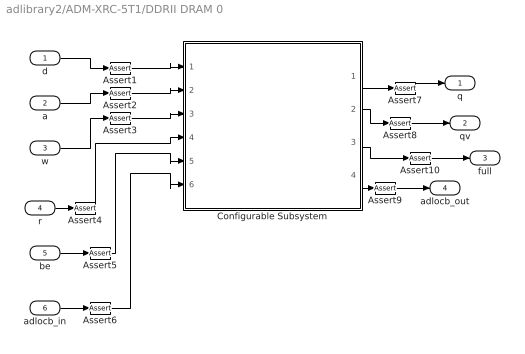
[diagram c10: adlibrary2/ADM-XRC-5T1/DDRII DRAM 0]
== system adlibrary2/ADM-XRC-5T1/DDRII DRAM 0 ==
  d : Inport
  a : Inport  Port=2
  w : Inport  Port=3
  r : Inport  Port=4
  be : Inport  Port=5
  adlocb_in : Inport  Port=6
  Assert{1..10} (10 alike) : xbsIndex_r4/Assert  assert_type=off  type_source=Explicitly  arith_type="Signed  (2's comp)"  n_bits=16  bin_pt=14  assert_rate=on  rate_source=Explicitly  period=ad_get_simulink_period  output_port=on  block_type=assert
  Configurable Subsystem : Subsystem  Tag=configX  BlockChoice=DDRII DRAM Simulation
  q : Outport
  qv : Outport  Port=2
  full : Outport  Port=3
  adlocb_out : Outport  Port=4
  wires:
  Configurable Subsystem/3(full) -> Assert10/1
  Assert10/1 -> full/1
  Configurable Subsystem/1(q) -> Assert7/1
  d/1 -> Assert1/1
  a/1 -> Assert2/1
  w/1 -> Assert3/1
  r/1 -> Assert4/1
  be/1 -> Assert5/1
  adlocb_in/1 -> Assert6/1
  Configurable Subsystem/4(adlocb_out) -> Assert9/1
  Configurable Subsystem/2(qv) -> Assert8/1
  Assert1/1 -> Configurable Subsystem/1(d)
  Assert2/1 -> Configurable Subsystem/2(a)
  Assert3/1 -> Configurable Subsystem/3(w)
  Assert4/1 -> Configurable Subsystem/4(r)
  Assert5/1 -> Configurable Subsystem/5(be)
  Assert6/1 -> Configurable Subsystem/6(adlocb_in)
  Assert7/1 -> q/1
  Assert8/1 -> qv/1
  Assert9/1 -> adlocb_out/1

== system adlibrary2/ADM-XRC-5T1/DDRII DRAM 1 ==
  d : Inport
  a : Inport  Port=2
  w : Inport  Port=3
  r : Inport  Port=4
  be : Inport  Port=5
  adlocb_in : Inport  Port=6
  Assert{1..10} (10 alike) : xbsIndex_r4/Assert  assert_type=off  type_source=Explicitly  arith_type="Signed  (2's comp)"  n_bits=16  bin_pt=14  assert_rate=on  rate_source=Explicitly  period=ad_get_simulink_period  output_port=on  block_type=assert
  Configurable Subsystem : Subsystem  Tag=configX  BlockChoice=DDRII DRAM Simulation
  q : Outport
  qv : Outport  Port=2
  full : Outport  Port=3
  adlocb_out : Outport  Port=4
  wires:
  Assert9/1 -> adlocb_out/1
  Assert8/1 -> qv/1
  Assert7/1 -> q/1
  Assert6/1 -> Configurable Subsystem/6(adlocb_in)
  Assert5/1 -> Configurable Subsystem/5(be)
  Assert3/1 -> Configurable Subsystem/3(w)
  Assert2/1 -> Configurable Subsystem/2(a)
  Assert1/1 -> Configurable Subsystem/1(d)
  adlocb_in/1 -> Assert6/1
  be/1 -> Assert5/1
  r/1 -> Assert4/1
  w/1 -> Assert3/1
  a/1 -> Assert2/1
  d/1 -> Assert1/1
  Assert10/1 -> full/1
  Assert4/1 -> Configurable Subsystem/4(r)
  Configurable Subsystem/4(adlocb_out) -> Assert9/1
  Configurable Subsystem/3(full) -> Assert10/1
  Configurable Subsystem/2(qv) -> Assert8/1
  Configurable Subsystem/1(q) -> Assert7/1

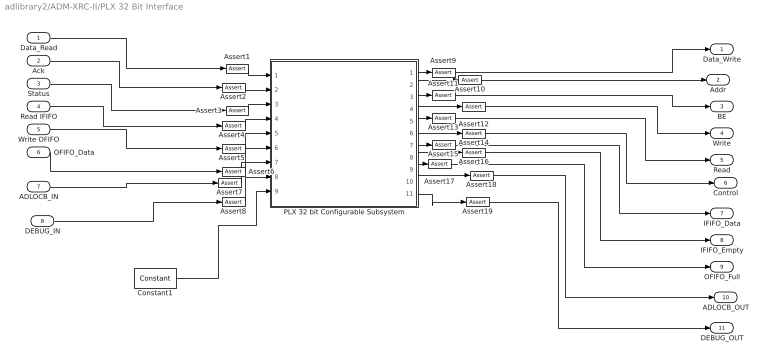
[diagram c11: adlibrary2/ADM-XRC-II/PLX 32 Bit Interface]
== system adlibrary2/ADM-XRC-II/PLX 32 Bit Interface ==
  Data_Read : Inport
  Ack : Inport  Port=2
  Status : Inport  Port=3
  Read IFIFO : Inport  Port=4
  Write OFIFO : Inport  Port=5
  OFIFO_Data : Inport  Port=6
  ADLOCB_IN : Inport  Port=7
  DEBUG_IN : Inport  Port=8
  Assert{1..19} (19 alike) : xbsIndex_r4/Assert  assert_type=off  type_source=Explicitly  arith_type="Signed  (2's comp)"  n_bits=16  bin_pt=14  assert_rate=on  rate_source=Explicitly  period=ad_get_simulink_period  output_port=on  block_type=assert
  Constant1 : xbsIndex_r4/Constant  arith_type=Boolean  const=sstep_clk_sel_default  n_bits=16  bin_pt=14  explicit_period=on  period=ad_get_simulink_period  equ=P=C  opselect=C  inp2=PCIN>>17  opr=+  inp1=P  carry=CIN  dbl_ovrd=off  block_type=constant
  PLX 32 bit Configurable Subsystem : Subsystem  Tag=configX  BlockChoice=PLX 32Bit Simulation  mask{program=program, clock_ratio=clock_ratio}
      mask prompts: program "Local Bus Script Program"; clock_ratio "Clock Ratio"
  Data_Write : Outport
  Addr : Outport  Port=2
  BE : Outport  Port=3
  Write : Outport  Port=4
  Read : Outport  Port=5
  Control : Outport  Port=6
  IFIFO_Data : Outport  Port=7
  IFIFO_Empty : Outport  Port=8
  OFIFO_Full : Outport  Port=9
  ADLOCB_OUT : Outport  Port=10
  DEBUG_OUT : Outport  Port=11
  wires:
  PLX 32 bit Configurable Subsystem/1(Data_Write) -> Assert9/1
  PLX 32 bit Configurable Subsystem/2(Addr) -> Assert10/1
  PLX 32 bit Configurable Subsystem/4(Write) -> Assert12/1
  PLX 32 bit Configurable Subsystem/6(Control) -> Assert14/1
  PLX 32 bit Configurable Subsystem/7(IFIFO_Data) -> Assert15/1
  PLX 32 bit Configurable Subsystem/8(IFIFO_Empty) -> Assert16/1
  PLX 32 bit Configurable Subsystem/9(OFIFO_Full) -> Assert17/1
  PLX 32 bit Configurable Subsystem/3(BE) -> Assert11/1
  PLX 32 bit Configurable Subsystem/10(ADLOCB_OUT) -> Assert18/1
  Data_Read/1 -> Assert1/1
  Ack/1 -> Assert2/1
  Status/1 -> Assert3/1
  Read IFIFO/1 -> Assert4/1
  Write OFIFO/1 -> Assert5/1
  OFIFO_Data/1 -> Assert6/1
  ADLOCB_IN/1 -> Assert7/1
  PLX 32 bit Configurable Subsystem/5(Read) -> Assert13/1
  Assert1/1 -> PLX 32 bit Configurable Subsystem/1(Data_Read)
  Assert2/1 -> PLX 32 bit Configurable Subsystem/2(Ack)
  Assert3/1 -> PLX 32 bit Configurable Subsystem/3(Status)
  Assert4/1 -> PLX 32 bit Configurable Subsystem/4(Read IFIFO)
  Assert5/1 -> PLX 32 bit Configurable Subsystem/5(Write OFIFO)
  Assert6/1 -> PLX 32 bit Configurable Subsystem/6(OFIFO_Data)
  Assert7/1 -> PLX 32 bit Configurable Subsystem/7(ADLOCB_IN)
  Assert9/1 -> Data_Write/1
  Assert10/1 -> Addr/1
  Assert11/1 -> BE/1
  Assert12/1 -> Write/1
  Assert13/1 -> Read/1
  Assert14/1 -> Control/1
  Assert15/1 -> IFIFO_Data/1
  Assert16/1 -> IFIFO_Empty/1
  Assert17/1 -> OFIFO_Full/1
  Assert18/1 -> ADLOCB_OUT/1
  DEBUG_IN/1 -> Assert8/1
  PLX 32 bit Configurable Subsystem/11(DEBUG_OUT) -> Assert19/1
  Assert19/1 -> DEBUG_OUT/1
  Assert8/1 -> PLX 32 bit Configurable Subsystem/8(DEBUG_IN)
  Constant1/1 -> PLX 32 bit Configurable Subsystem/9(sstep_clk_sel_default)

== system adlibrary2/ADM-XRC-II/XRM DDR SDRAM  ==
  cache_data_in : Inport
  cache_addr : Inport  Port=2
  cache_write : Inport  Port=3
  ddr_page : Inport  Port=4
  ddr_addr : Inport  Port=5
  ddr_read : Inport  Port=6
  ddr_write : Inport  Port=7
  Assert{1..9} (9 alike) : xbsIndex_r4/Assert  assert_type=off  type_source=Explicitly  arith_type="Signed  (2's comp)"  n_bits=16  bin_pt=14  assert_rate=on  rate_source=Explicitly  period=ad_get_simulink_period  output_port=on  block_type=assert
  Configurable Subsystem : Subsystem  Tag=configX  BlockChoice=DDR SDRAM 64bit Simulation
  cache_data_out : Outport
  ddr_busy : Outport  Port=2
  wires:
  cache_data_in/1 -> Assert1/1
  cache_addr/1 -> Assert2/1
  cache_write/1 -> Assert3/1
  ddr_page/1 -> Assert4/1
  ddr_addr/1 -> Assert5/1
  ddr_read/1 -> Assert6/1
  ddr_write/1 -> Assert7/1
  Configurable Subsystem/1(cache_data_out) -> Assert8/1
  Configurable Subsystem/2(ddr_busy) -> Assert9/1
  Assert1/1 -> Configurable Subsystem/1(cache_data_in)
  Assert2/1 -> Configurable Subsystem/2(cache_addr)
  Assert3/1 -> Configurable Subsystem/3(cache_write)
  Assert4/1 -> Configurable Subsystem/4(ddr_page)
  Assert5/1 -> Configurable Subsystem/5(ddr_addr)
  Assert6/1 -> Configurable Subsystem/6(ddr_read)
  Assert7/1 -> Configurable Subsystem/7(ddr_write)
  Assert8/1 -> cache_data_out/1
  Assert9/1 -> ddr_busy/1

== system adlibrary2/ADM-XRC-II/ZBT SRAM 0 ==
  d : Inport
  a : Inport  Port=2
  w : Inport  Port=3
  r : Inport  Port=4
  be : Inport  Port=5
  adlocb_in : Inport  Port=6
  Assert{,1..8} (9 alike) : xbsIndex_r4/Assert  assert_type=off  type_source=Explicitly  arith_type="Signed  (2's comp)"  n_bits=16  bin_pt=14  assert_rate=on  rate_source=Explicitly  period=ad_get_simulink_period  output_port=on  block_type=assert
  Configurable Subsystem : Subsystem  Tag=configX  BlockChoice=ZBT SRAM 32Bit Simulation
  q : Outport
  qv : Outport  Port=2
  adlocb_out : Outport  Port=3
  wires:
  d/1 -> Assert/1
  a/1 -> Assert1/1
  w/1 -> Assert2/1
  r/1 -> Assert4/1
  be/1 -> Assert3/1
  adlocb_in/1 -> Assert5/1
  Configurable Subsystem/1(q) -> Assert6/1
  Configurable Subsystem/2(qv) -> Assert7/1
  Configurable Subsystem/3(adlocb_out) -> Assert8/1
  Assert/1 -> Configurable Subsystem/1(d)
  Assert1/1 -> Configurable Subsystem/2(a)
  Assert2/1 -> Configurable Subsystem/3(w)
  Assert4/1 -> Configurable Subsystem/4(r)
  Assert3/1 -> Configurable Subsystem/5(be)
  Assert5/1 -> Configurable Subsystem/6(adlocb_in)
  Assert8/1 -> adlocb_out/1
  Assert7/1 -> qv/1
  Assert6/1 -> q/1

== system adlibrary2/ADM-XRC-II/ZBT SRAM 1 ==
  d : Inport
  a : Inport  Port=2
  w : Inport  Port=3
  r : Inport  Port=4
  be : Inport  Port=5
  adlocb_in : Inport  Port=6
  Assert{,1..8} (9 alike) : xbsIndex_r4/Assert  assert_type=off  type_source=Explicitly  arith_type="Signed  (2's comp)"  n_bits=16  bin_pt=14  assert_rate=on  rate_source=Explicitly  period=ad_get_simulink_period  output_port=on  block_type=assert
  Configurable Subsystem : Subsystem  Tag=configX  BlockChoice=ZBT SRAM 32Bit Simulation
  q : Outport
  qv : Outport  Port=2
  adlocb_out : Outport  Port=3
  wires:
  Configurable Subsystem/3(adlocb_out) -> Assert8/1
  Configurable Subsystem/2(qv) -> Assert7/1
  Configurable Subsystem/1(q) -> Assert6/1
  adlocb_in/1 -> Assert5/1
  be/1 -> Assert4/1
  r/1 -> Assert3/1
  w/1 -> Assert2/1
  a/1 -> Assert1/1
  d/1 -> Assert/1
  Assert/1 -> Configurable Subsystem/1(d)
  Assert1/1 -> Configurable Subsystem/2(a)
  Assert2/1 -> Configurable Subsystem/3(w)
  Assert3/1 -> Configurable Subsystem/4(r)
  Assert4/1 -> Configurable Subsystem/5(be)
  Assert5/1 -> Configurable Subsystem/6(adlocb_in)
  Assert6/1 -> q/1
  Assert7/1 -> qv/1
  Assert8/1 -> adlocb_out/1

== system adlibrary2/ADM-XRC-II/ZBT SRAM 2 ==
  d : Inport
  a : Inport  Port=2
  w : Inport  Port=3
  r : Inport  Port=4
  be : Inport  Port=5
  adlocb_in : Inport  Port=6
  Assert{,1..8} (9 alike) : xbsIndex_r4/Assert  assert_type=off  type_source=Explicitly  arith_type="Signed  (2's comp)"  n_bits=16  bin_pt=14  assert_rate=on  rate_source=Explicitly  period=ad_get_simulink_period  output_port=on  block_type=assert
  Configurable Subsystem : Subsystem  Tag=configX  BlockChoice=ZBT SRAM 32Bit Simulation
  q : Outport
  qv : Outport  Port=2
  adlocb_out : Outport  Port=3
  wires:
  Configurable Subsystem/3(adlocb_out) -> Assert8/1
  Configurable Subsystem/2(qv) -> Assert7/1
  Configurable Subsystem/1(q) -> Assert6/1
  adlocb_in/1 -> Assert5/1
  be/1 -> Assert4/1
  r/1 -> Assert3/1
  w/1 -> Assert2/1
  a/1 -> Assert1/1
  d/1 -> Assert/1
  Assert/1 -> Configurable Subsystem/1(d)
  Assert1/1 -> Configurable Subsystem/2(a)
  Assert2/1 -> Configurable Subsystem/3(w)
  Assert3/1 -> Configurable Subsystem/4(r)
  Assert4/1 -> Configurable Subsystem/5(be)
  Assert5/1 -> Configurable Subsystem/6(adlocb_in)
  Assert6/1 -> q/1
  Assert7/1 -> qv/1
  Assert8/1 -> adlocb_out/1

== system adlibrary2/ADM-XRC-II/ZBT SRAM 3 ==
  d : Inport
  a : Inport  Port=2
  w : Inport  Port=3
  r : Inport  Port=4
  be : Inport  Port=5
  adlocb_in : Inport  Port=6
  Assert{,1..8} (9 alike) : xbsIndex_r4/Assert  assert_type=off  type_source=Explicitly  arith_type="Signed  (2's comp)"  n_bits=16  bin_pt=14  assert_rate=on  rate_source=Explicitly  period=ad_get_simulink_period  output_port=on  block_type=assert
  Configurable Subsystem : Subsystem  Tag=configX  BlockChoice=ZBT SRAM 32Bit Simulation
  q : Outport
  qv : Outport  Port=2
  adlocb_out : Outport  Port=3
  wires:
  Configurable Subsystem/3(adlocb_out) -> Assert7/1
  Configurable Subsystem/2(qv) -> Assert6/1
  Configurable Subsystem/1(q) -> Assert8/1
  adlocb_in/1 -> Assert5/1
  be/1 -> Assert4/1
  r/1 -> Assert3/1
  w/1 -> Assert2/1
  a/1 -> Assert1/1
  d/1 -> Assert/1
  Assert/1 -> Configurable Subsystem/1(d)
  Assert1/1 -> Configurable Subsystem/2(a)
  Assert2/1 -> Configurable Subsystem/3(w)
  Assert3/1 -> Configurable Subsystem/4(r)
  Assert4/1 -> Configurable Subsystem/5(be)
  Assert5/1 -> Configurable Subsystem/6(adlocb_in)
  Assert8/1 -> q/1
  Assert6/1 -> qv/1
  ? -> adlocb_out/1

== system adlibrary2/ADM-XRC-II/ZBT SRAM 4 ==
  d : Inport
  a : Inport  Port=2
  w : Inport  Port=3
  r : Inport  Port=4
  be : Inport  Port=5
  adlocb_in : Inport  Port=6
  Assert{,1..8} (9 alike) : xbsIndex_r4/Assert  assert_type=off  type_source=Explicitly  arith_type="Signed  (2's comp)"  n_bits=16  bin_pt=14  assert_rate=on  rate_source=Explicitly  period=ad_get_simulink_period  output_port=on  block_type=assert
  Configurable Subsystem : Subsystem  Tag=configX  BlockChoice=ZBT SRAM 32Bit Simulation
  q : Outport
  qv : Outport  Port=2
  adlocb_out : Outport  Port=3
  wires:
  Configurable Subsystem/3(adlocb_out) -> Assert8/1
  Configurable Subsystem/2(qv) -> Assert7/1
  Configurable Subsystem/1(q) -> Assert6/1
  adlocb_in/1 -> Assert5/1
  be/1 -> Assert4/1
  r/1 -> Assert3/1
  w/1 -> Assert2/1
  a/1 -> Assert1/1
  d/1 -> Assert/1
  Assert/1 -> Configurable Subsystem/1(d)
  Assert1/1 -> Configurable Subsystem/2(a)
  Assert2/1 -> Configurable Subsystem/3(w)
  Assert3/1 -> Configurable Subsystem/4(r)
  Assert4/1 -> Configurable Subsystem/5(be)
  Assert5/1 -> Configurable Subsystem/6(adlocb_in)
  Assert6/1 -> q/1
  Assert7/1 -> qv/1
  Assert8/1 -> adlocb_out/1

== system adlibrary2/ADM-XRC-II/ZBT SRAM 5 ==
  d : Inport
  a : Inport  Port=2
  w : Inport  Port=3
  r : Inport  Port=4
  be : Inport  Port=5
  adlocb_in : Inport  Port=6
  Assert{,1..8} (9 alike) : xbsIndex_r4/Assert  assert_type=off  type_source=Explicitly  arith_type="Signed  (2's comp)"  n_bits=16  bin_pt=14  assert_rate=on  rate_source=Explicitly  period=ad_get_simulink_period  output_port=on  block_type=assert
  Configurable Subsystem : Subsystem  Tag=configX  BlockChoice=ZBT SRAM 32Bit Simulation
  q : Outport
  qv : Outport  Port=2
  adlocb_out : Outport  Port=3
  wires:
  Configurable Subsystem/3(adlocb_out) -> Assert8/1
  Configurable Subsystem/2(qv) -> Assert7/1
  Configurable Subsystem/1(q) -> Assert6/1
  adlocb_in/1 -> Assert5/1
  be/1 -> Assert4/1
  r/1 -> Assert3/1
  w/1 -> Assert2/1
  a/1 -> Assert1/1
  d/1 -> Assert/1
  Assert/1 -> Configurable Subsystem/1(d)
  Assert1/1 -> Configurable Subsystem/2(a)
  Assert2/1 -> Configurable Subsystem/3(w)
  Assert3/1 -> Configurable Subsystem/4(r)
  Assert4/1 -> Configurable Subsystem/5(be)
  Assert5/1 -> Configurable Subsystem/6(adlocb_in)
  Assert6/1 -> q/1
  Assert7/1 -> qv/1
  Assert8/1 -> adlocb_out/1
